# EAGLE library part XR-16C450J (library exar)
UART
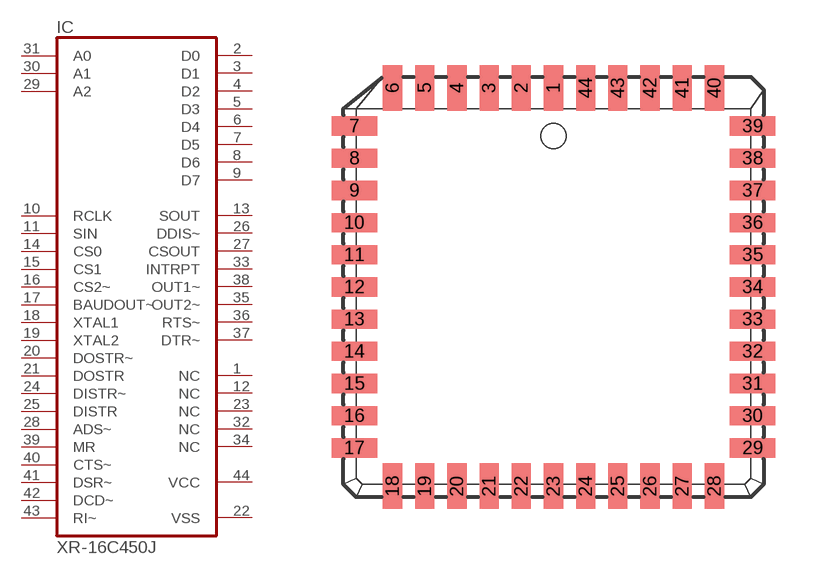
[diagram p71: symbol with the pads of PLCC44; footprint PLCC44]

Designator prefix IC

## XR-16C450J (MF: TEXAS INSTRUMENTS; MPN: TL16C450FNR; OC_FARNELL: unknown; OC_NEWARK: 76C9161)  [PLCC44]
1  NC  nc
2  D0
3  D1
4  D2
5  D3
6  D4
7  D5
8  D6
9  D7
10  RCLK  in
11  SIN  in
12  NC  nc
13  SOUT  out
14  CS0  in
15  CS1  in
16  CS2~  in
17  BAUDOUT~  in
18  XTAL1  in
19  XTAL2  in
20  DOSTR~  in
21  DOSTR  in
22  VSS  pwr
23  NC  nc
24  DISTR~  in
25  DISTR  in
26  DDIS~  out
27  CSOUT  out
28  ADS~  in
29  A2  in
30  A1  in
31  A0  in
32  NC  nc
33  INTRPT  out
34  NC  nc
35  OUT2~  out
36  RTS~  out
37  DTR~  out
38  OUT1~  out
39  MR  in
40  CTS~  in
41  DSR~  in
42  DCD~  in
43  RI~  in
44  VCC  pwr

## Footprint PLCC44 (pad centres in mm)
Plastic Leaded Chip Carrier
smd 0.76 x 1.8: 1 0,7.86; 2 -1.27,7.86; 3 -2.54,7.86; 4 -3.81,7.86; 5 -5.08,7.86; 6 -6.35,7.86; 18 -6.35,-7.86; 19 -5.08,-7.86; 20 -3.81,-7.86; 21 -2.54,-7.86; 22 -1.27,-7.86; 23 0,-7.86; 24 1.27,-7.86; 25 2.54,-7.86; 26 3.81,-7.86; 27 5.08,-7.86; 28 6.35,-7.86; 40 6.35,7.86; 41 5.08,7.86; 42 3.81,7.86; 43 2.54,7.86; 44 1.27,7.86
smd 1.8 x 0.76: 7 -7.86,6.35; 8 -7.86,5.08; 9 -7.86,3.81; 10 -7.86,2.54; 11 -7.86,1.27; 12 -7.86,0; 13 -7.86,-1.27; 14 -7.86,-2.54; 15 -7.86,-3.81; 16 -7.86,-5.08; 17 -7.86,-6.35; 29 7.86,-6.35; 30 7.86,-5.08; 31 7.86,-3.81; 32 7.86,-2.54; 33 7.86,-1.27; 34 7.86,0; 35 7.86,1.27; 36 7.86,2.54; 37 7.86,3.81; 38 7.86,5.08; 39 7.86,6.35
